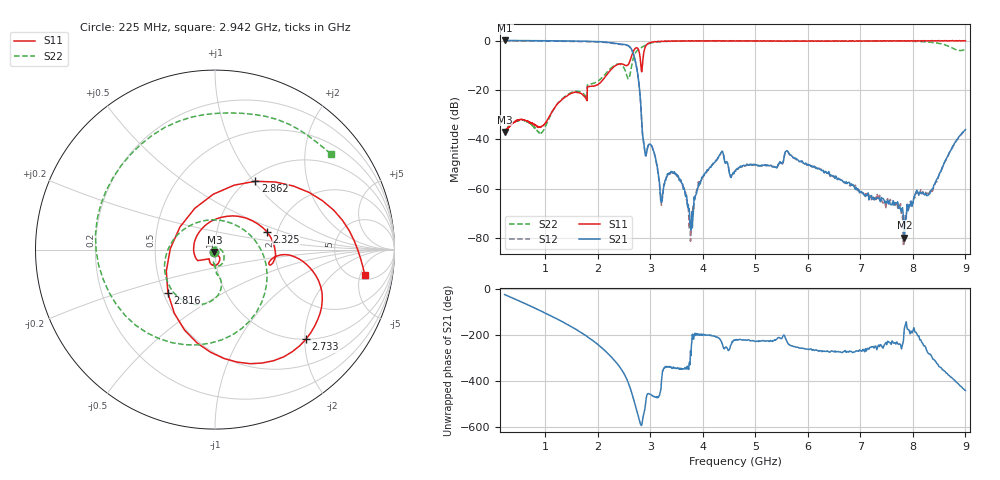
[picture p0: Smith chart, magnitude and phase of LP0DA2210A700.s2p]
!Agilent Technologies,E8358A,US41080443,A.07.50.56
!Agilent E8358A: A.07.50.56
!Date: Wednesday, May 04, 2016 15:20:48
!Correction: S11(Full 2 Port(1,2))
!S21(Full 2 Port(1,2))
!S12(Full 2 Port(1,2))
!S22(Full 2 Port(1,2))
!S2P File: Measurements: S11, S21, S12, S22:Log Frequency Sweep
# Hz S  dB  R 50
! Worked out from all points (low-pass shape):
!   1601 points, 225 MHz to 9 GHz, reference 50 ohm
!   highest |S21| = 0.03 dB at 233.5 MHz (marker M1); lowest = -79.9 dB at 7.837 GHz (marker M2)
!   |S21| within 3 dB of the highest: start of sweep to 2.626 GHz
!   lowest |S11| = -37.0 dB at 225 MHz (marker M3), VSWR 1.03, Z = 49.7 - j1.36 ohm
!   |S11| at or under -10 dB: start of sweep to 2.348 GHz; 2.517 GHz to 2.568 GHz (50.84 MHz wide, 2 % of centre); 2.82 GHz to 2.849 GHz (29.15 MHz wide, 1.03 % of centre)
!   |S22| runs from -37.6 to -0.1 dB; largest |S21 - S12| = 0.019
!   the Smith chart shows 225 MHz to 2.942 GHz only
!   S11 on the Smith chart (normalised r, x): 225 MHz: 0.99, -0.03; 2.325 GHz: 1.75, +0.39; 2.733 GHz: 1.00, -2.03; 2.816 GHz: 0.53, -0.29; 2.862 GHz: 1.08, +1.02; 2.942 GHz: 6.01, -5.97
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2.25e8  -37.02 -103.6  0.03 -22.7  -0.12 -22.6  -36.78 -120.3
2.33455e8  -36.69 -103.8  0.03 -23.6  -0.13 -23.4  -36.61 -121.3
9.817598e8  -33.96 -77.3  -0.08 -101.3  -0.23 -101.1  -35.84 46.5
1.687749e9  -21.53 -105.9  -0.24 171.2  -0.39 171.3  -21.00 -89.2
2.067384e9  -16.64 109.7  -0.50 107.0  -0.66 107.1  -15.36 -79.4
2.325342e9  -10.32 19.1  -1.12 48.2  -1.28 48.4  -10.01 -105.5
2.49187e9  -9.72 -14.4  -1.54 -4.3  -1.71 -4.4  -10.89 -167.5
2.603454e9  -8.77 -4.8  -2.44 -61.1  -2.58 -61.0  -14.76 45.3
2.732605e9  -2.96 -44.6  -10.18 -159.7  -10.30 -159.7  -4.45 -129.1
2.815747e9  -8.93 -137.2  -25.30 131.3  -25.48 131.5  -3.08 138.2
2.861558e9  -7.09 59.5  -39.66 164.2  -39.79 163.7  -2.45 94.4
2.941833e9  -1.45 -9.6  -43.86 -97.0  -44.01 -96.8  -1.54 39.6
3.152512e9  -0.33 -53.6  -54.24 -108.4  -54.18 -106.1  -0.49 -29.8
3.513316e9  -0.24 -80.3  -54.86 16.1  -55.20 14.4  -0.24 -74.1
3.764921e9  -0.22 -91.5  -74.67 92.3  -81.39 57.8  -0.19 -91.4
4.303586e9  -0.12 -107.2  -47.10 147.5  -47.05 148.6  -0.12 -118.8
4.622431e9  -0.17 -114.9  -52.84 140.6  -53.01 139.6  -0.14 -133.2
6.081681e9  -0.15 -153.5  -51.35 94.1  -51.00 97.2  -0.22 151.7
7.553438e9  -0.21 173.4  -65.15 128.1  -65.23 133.1  -0.12 97.1
7.837278e9  -0.07 169.2  -79.88 -170.3  -81.68 -178.2  -0.22 86.6
8.614261e9  -0.03 163.4  -48.88 1.9  -49.00 -0.7  -1.80 18.1
9e9  -0.08 160.8  -36.12 -80.4  -36.35 -80.5  -3.53 -134.0
